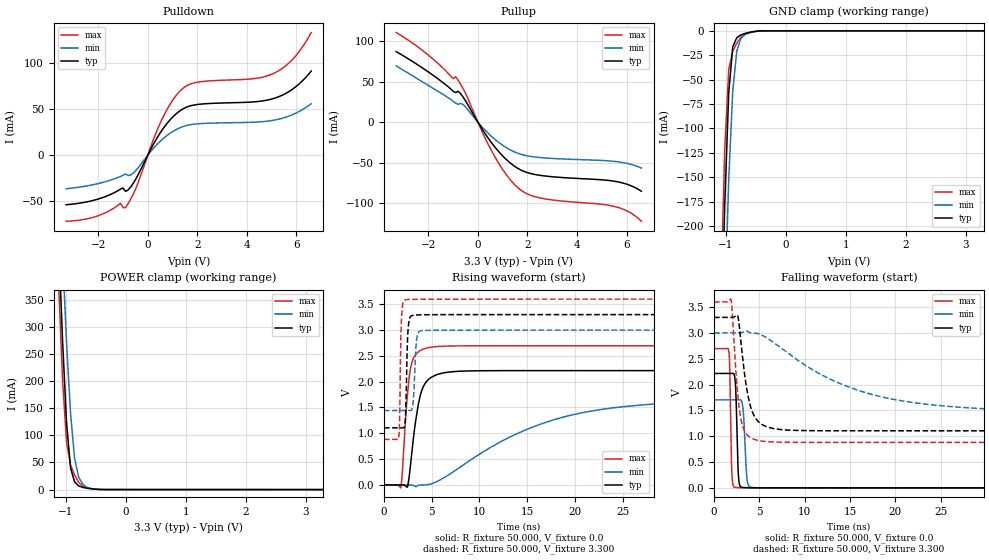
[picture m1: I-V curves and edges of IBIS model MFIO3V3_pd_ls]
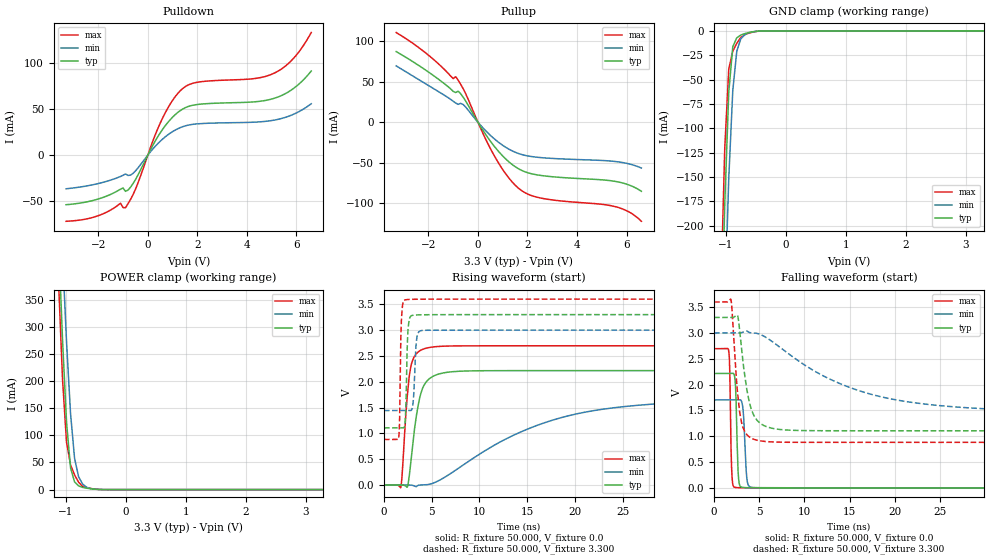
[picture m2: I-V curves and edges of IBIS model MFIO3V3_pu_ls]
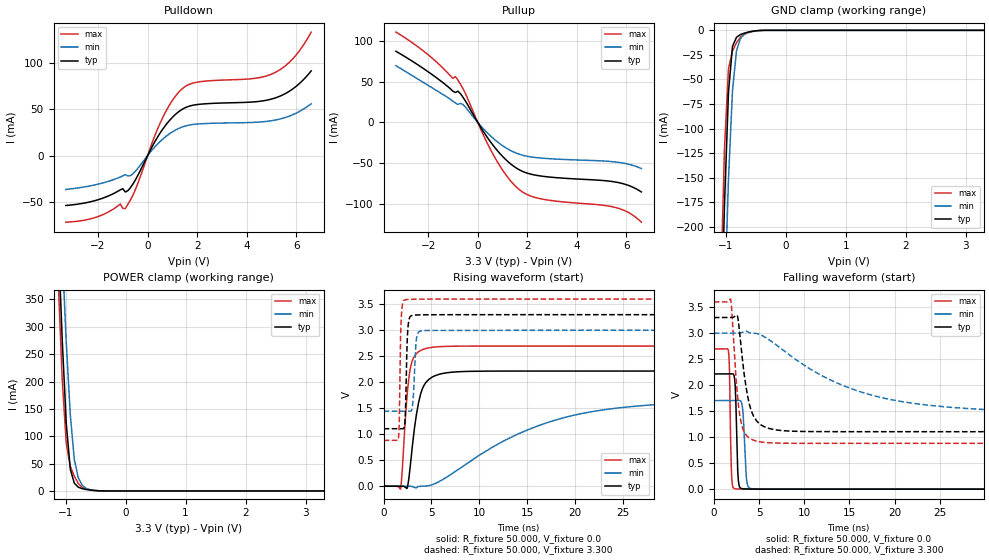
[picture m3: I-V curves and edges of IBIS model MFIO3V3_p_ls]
| IBIS file lpc55s1x_vfbga98.ibs
[IBIS Ver]   5.0
[File name]   lpc55s1x_vfbga98.ibs
[File Rev]   1.0
[Date]   June 18,2020
[Notes]   Rev History
|   1.0  initial release
[Disclaimer]   The model given below represents a 98-pin package.
[Copyright]   Copyright NXP 2020
|   Component lpc55s1x:vfbga98
[Component] lpc55s1x
[Manufacturer] NXP
[Package]
|   typ   min   max
R_pkg   0.13061   0.065508   0.30829
L_pkg   2.046e-9   9.939e-10   5.651e-9
C_pkg   3.491e-13   2.146e-13   5.779e-13
[Pin]   Signal_name   model_name   R_pin   L_pin   C_pin
N13   VBAT_DCDC   POWER   NA   NA   NA
M13   VBAT_PMU   POWER   NA   NA   NA
N8   VBUS   POWER   NA   NA   NA
A9   VDD   POWER   NA   NA   NA
A5   VDD   POWER   NA   NA   NA
M1   VDD   POWER   NA   NA   NA
A13   VDD   POWER   NA   NA   NA
G2   VDDA   POWER   NA   NA   NA
N7   USB1_3V3   POWER   NA   NA   NA
A3   USB0_3V3   POWER   NA   NA   NA
M9   VDD_PMU   POWER   NA   NA   NA
H1   VREFN   NC   NA   NA   NA
G1   VREFP   NC   NA   NA   NA
N6   USB1_DM   NC   0.11669   1.732e-9   2.843e-13
M6   USB1_DP   NC   0.11608   1.667e-9   2.908e-13
N9   FB   NC   0.1161   1.684e-9   2.591e-13
N11   LX   NC   0.065508   1.382e-9   3.314e-13
L12   P0_0   gpio3v3   0.14455   2.198e-9   3.521e-13
F5   P0_1   gpio3v3   0.090747   1.591e-9   4.4e-13
B11   P0_2   gpio3v3   0.13207   1.835e-9   3.536e-13
F8   P0_3   gpio3v3   0.10051   1.437e-9   4.428e-13
E7   P0_4   gpio3v3   0.07496   1.173e-9   3.73e-13
A7   P0_5   gpio3v3   0.14141   2.213e-9   2.521e-13
B7   P0_6   gpio3v3   0.10225   1.431e-9   2.556e-13
G5   P0_7   gpio3v3   0.14307   2.547e-9   5.485e-13
M2   P0_8   gpio3v3   0.13069   1.904e-9   2.997e-13
L13   P0_9   gpio3v3   0.16996   2.85e-9   3.914e-13
F2   P0_10   gpio3v3   0.1455   2.479e-9   3.552e-13
F1   P0_11   gpio3v3   0.12654   1.782e-9   2.328e-13
E2   P0_12   gpio3v3   0.12249   2.232e-9   2.882e-13
C12   P0_13   iicgpio3v3  0.13173   2.058e-9   2.548e-13
C13   P0_14   iicgpio3v3  0.14686   2.267e-9   2.614e-13
L2   P0_15   gpio3v3   0.11536   1.578e-9   3.074e-13
J2   P0_16   gpio3v3   0.16378   2.774e-9   3.403e-13
G3   P0_17   gpio3v3   0.076051   1.338e-9   3.659e-13
H9   P0_18   gpio3v3   0.099545   1.572e-9   4.786e-13
E6   P0_19   gpio3v3   0.10118   1.907e-9   4.333e-13
B12   P0_20   gpio3v3   0.13506   2.134e-9   3.591e-13
A12   P0_21   gpio3v3   0.14732   2.073e-9   3.225e-13
E9   P0_22   gpio3v3   0.078558   9.939e-10   3.497e-13
J1   P0_23   gpio3v3   0.13644   1.839e-9   2.161e-13
E12   P0_24   gpio3v3   0.14263   2.181e-9   2.725e-13
A11   P0_25   gpio3v3   0.14798   2.102e-9   2.79e-13
H12   P0_26   gpio3v3   0.11228   1.606e-9   2.445e-13
N2   P0_27   gpio3v3   0.16245   2.487e-9   3.312e-13
F13   P0_28   gpio3v3   0.12376   1.834e-9   2.235e-13
H8   P0_29   gpio3v3   0.13203   2.551e-9   5.469e-13
E5   P0_30   gpio3v3   0.084435   1.283e-9   4.113e-13
L1   P0_31   gpio3v3   0.14669   2.123e-9   2.715e-13
E1   P1_0   gpio3v3   0.13529   2.048e-9   2.414e-13
G11   P1_1   gpio3v3   0.074092   1.205e-9   2.789e-13
G12   P1_2   gpio3v3   0.10494   1.512e-9   2.312e-13
G13   P1_3   gpio3v3   0.12602   1.85e-9   2.146e-13
B2   P1_4   gpio3v3   0.1228   1.733e-9   2.552e-13
M5   P1_5   gpio3v3   0.13163   1.821e-9   2.471e-13
H5   P1_6   gpio3v3   0.17302   2.947e-9   5.779e-13
J5   P1_7   gpio3v3   0.13225   2.135e-9   5.089e-13
A6   P1_8   gpio3v3   0.2994   5.534e-9   4.497e-13
C1   P1_9   gpio3v3   0.15079   2.581e-9   2.461e-13
J7   P1_10   gpio3v3   0.095691   1.435e-9   3.574e-13
G6   P1_11   gpio3v3   0.12438   2.138e-9   5.286e-13
F12   P1_12   gpio3v3   0.10269   1.43e-9   2.354e-13
B3   P1_13   gpio3v3   0.096086   1.515e-9   3.876e-13
L7   P1_14   gpio3v3   0.19623   3.642e-9   4.84e-13
B6   P1_15   gpio3v3   0.17552   2.69e-9   3.435e-13
C7   P1_16   gpio3v3   0.096915   1.392e-9   2.638e-13
J9   P1_17   gpio3v3   0.092963   1.486e-9   3.448e-13
G9   P1_18   gpio3v3   0.099814   1.421e-9   3.963e-13
H13   P1_19   gpio3v3   0.13318   2.11e-9   2.391e-13
C2   P1_20   gpio3v3   0.12316   2.129e-9   3.37e-13
M7   P1_21   gpio3v3   0.11945   2.176e-9   4.385e-13
M8   P1_22   gpio3v3   0.10948   1.392e-9   2.932e-13
J8   P1_23   gpio3v3   0.075093   9.959e-10   3.672e-13
F6   P1_24   gpio3v3   0.13859   2.139e-9   5.025e-13
B8   P1_25   gpio3v3   0.21198   3.592e-9   3.673e-13
E13   P1_26   gpio3v3   0.12693   1.882e-9   2.48e-13
E8   P1_27   gpio3v3   0.097026   1.482e-9   4.012e-13
A8   P1_28   gpio3v3   0.30829   5.651e-9   4.711e-13
G8   P1_29   gpio3v3   0.1184   1.994e-9   5.418e-13
F9   P1_30   gpio3v3   0.096855   1.515e-9   4.153e-13
H6   P1_31   gpio3v3   0.15561   2.896e-9   5.731e-13
J6   RESETN   gpio3v3   0.11246   1.658e-9   3.351e-13
A1   USB0_DM   NC   0.18721   2.704e-9   3.289e-13
A2   USB0_DP   NC   0.17884   2.424e-9   3.329e-13
J12   XTAL32K_N   NC   0.11929   1.659e-9   2.629e-13
J13   XTAL32K_P   NC   0.14517   1.945e-9   2.651e-13
M3   XTAL32M_N   NC   0.13348   1.673e-9   4.297e-13
N3   XTAL32M_P   NC   0.15113   2.064e-9   4.226e-13
B13   VSS   GND   NA   NA   NA
B9   VSS   GND   NA   NA   NA
B5   VSS   GND   NA   NA   NA
N1   VSS   GND   NA   NA   NA
H2   VSSA   GND   NA   NA   NA
N5   USB1_VSS   GND   NA   NA   NA
N12   VSS_DCDC   GND   NA   NA   NA
M12   VSS_DCDC   GND   NA   NA   NA
M11   VSS_PMU   GND   NA   NA   NA
B1   USB0_VSS   GND   NA   NA   NA
|   Model Selector
[Model Selector] gpio3v3
MFIO3V3_pd_hs  EPUN=1 EPD=1 EHS=1
MFIO3V3_pd_ls  EPUN=1 EPD=1 EHS=0
MFIO3V3_pu_hs  EPUN=0 EPD=0 EHS=1
MFIO3V3_pu_ls  EPUN=0 EPD=0 EHS=0
MFIO3V3_p_hs  EPUN=1 EPD=0 EHS=1
MFIO3V3_p_ls  EPUN=1 EPD=0 EHS=0
MFIO3V3_r_hs  EPUN=0 EPD=1 EHS=1
MFIO3V3_r_ls  EPUN=0 EPD=1 EHS=0
[Model Selector] iicgpio3v3
IIC3V3_pd_hs  EGP=1 EPUN=1 EPD=1 EHS=1
IIC3V3_pd_ls  EGP=1 EPUN=1 EPD=1 EHS=0
IIC3V3_p_hs  EGP=1 EPUN=1 EPD=0 EHS=1
IIC3V3_p_ls  EGP=1 EPUN=1 EPD=0 EHS=0
IIC3V3_pu_hs  EGP=1 EPUN=0 EPD=0 EHS=1
IIC3V3_pu_ls  EGP=1 EPUN=0 EPD=0 EHS=0
IIC3V3_r_hs  EGP=1 EPUN=0 EPD=1 EHS=1
IIC3V3_r_ls  EGP=1 EPUN=0 EPD=1 EHS=0
IIC3V3_pd_iic_hs  EGP=0 ECS=0 EPUN=1 EPD=1
IIC3V3_p_iic_hs  EGP=0 ECS=0 EPUN=1 EPD=0
IIC3V3_pu_iic_hs  EGP=0 ECS=0 EPUN=0 EPD=0
IIC3V3_r_iic_hs  EGP=0 ECS=0 EPUN=0 EPD=1
IIC3V3_pd_iic_pu_hs  EGP=0 ECS=1 EPUN=1 EPD=1  SSEL=1
IIC3V3_p_iic_pu_hs  EGP=0 ECS=1 EPUN=1 EPD=0  SSEL=1
IIC3V3_pu_iic_pu_hs  EGP=0 ECS=1 EPUN=0 EPD=0  SSEL=1
IIC3V3_r_iic_pu_hs  EGP=0 ECS=1 EPUN=0 EPD=1  SSEL=1
| Models and submodels in the file (24): MFIO3V3_pd_hs (I/O), MFIO3V3_pd_ls (I/O), MFIO3V3_pu_hs (I/O), MFIO3V3_pu_ls (I/O), MFIO3V3_p_hs (I/O), MFIO3V3_p_ls (I/O), MFIO3V3_r_hs (I/O), MFIO3V3_r_ls (I/O), IIC3V3_pd_hs (I/O), IIC3V3_pd_ls (I/O), IIC3V3_p_hs (I/O), IIC3V3_p_ls (I/O), IIC3V3_pu_hs (I/O), IIC3V3_pu_ls (I/O), IIC3V3_r_hs (I/O), IIC3V3_r_ls (I/O), IIC3V3_pd_iic_hs (I/O_open_drain), IIC3V3_p_iic_hs (I/O_open_drain), IIC3V3_pu_iic_hs (I/O_open_drain), IIC3V3_r_iic_hs (I/O_open_drain), IIC3V3_pd_iic_pu_hs (I/O_open_drain), IIC3V3_p_iic_pu_hs (I/O_open_drain), IIC3V3_pu_iic_pu_hs (I/O_open_drain), IIC3V3_r_iic_pu_hs (I/O_open_drain)
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|   Model MFIO3V3_pd_ls
[Model] MFIO3V3_pd_ls
Model_type I/O
Polarity   Non-Inverting
Enable   Active-Low
Vinl =  0.990V
Vinh =  2.310V
Vmeas =  1.650V
Cref =  0.0F
Rref =  100.000
Vref =  0.0V
C_comp   1.906pF   1.877pF   1.925pF
C_comp_pullup   1.141pF   1.113pF   1.145pF
C_comp_pulldown   0.641pF   0.601pF   0.647pF
[Model Spec]
Vinh   2.310V   2.100V   2.520V
Vinl   0.990V   0.900V   1.080V
Vmeas   1.650V   1.500V   1.800V
Vref   0.0V   0.0V   0.0V
Cref   0.0F   0.0F   0.0F
Rref   100.000   100.000   100.000
[Temperature Range]   25.000   0.125k   -40.000
[Voltage Range]   3.300V   3.000V   3.600V
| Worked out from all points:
|   slope of the pulldown table from 0 to 0.495 V, typ, clamps not added: 20.7 ohm
|   slope of the pullup table from 0 to 0.495 V, typ, clamps not added: 21.4 ohm
|   GND clamp passes 1 mA (typ) near -0.56 V on its own axis
|   POWER clamp passes 1 mA (typ) near -0.53 V on its own axis
|   rising waveform, R_fixture 50.000, V_fixture 0.0: 20-80 % time 1.05ns typ, 11.9ns min, 670ps max; typ from 0 V to 2.21 V
|   rising waveform, R_fixture 50.000, V_fixture 3.300: 20-80 % time 176ps typ, 234ps min, 146ps max; typ from 1.1 V to 3.3 V
|   falling waveform, R_fixture 50.000, V_fixture 0.0: 20-80 % time 203ps typ, 279ps min, 162ps max; typ from 2.21 V to 0 V
|   falling waveform, R_fixture 50.000, V_fixture 3.300: 20-80 % time 1.13ns typ, 11.2ns min, 744ps max; typ from 3.3 V to 1.1 V
[Pulldown]
|Voltage   I(typ)   I(min)   I(max)
-3.3V     -53.7mA    -36.43mA   -71.67mA
-2.1V     -48.29mA   -31.37mA   -66.51mA
-1.1V     -36.82mA   -23.05mA   -52.1mA
-900mV    -39.2mA    -20.39mA   -56.91mA
-600mV    -30.96mA   -19.83mA   -42.97mA
600mV     28.07mA    17.5mA     40.4mA
1V        41.17mA    25.53mA    59.41mA
1.4V      49.87mA    30.79mA    72.04mA
2V        54.93mA    33.94mA    79.03mA
5V        60.84mA    37.53mA    87.68mA
5.9V      72.62mA    44.52mA    105.4mA
6.6V      91.19mA    55.78mA    132.9mA
[Pullup]
|Voltage   I(typ)   I(min)   I(max)
-3.3V     87.16mA    69.54mA    110.7mA
-2.1V     64.12mA    47.22mA    85.31mA
-1V       38.1mA     25.85mA    53.88mA
-900mV    36.64mA    23.75mA    56.16mA
-800mV    38.25mA    22.02mA    51.93mA
-600mV    31.06mA    21.93mA    41.58mA
700mV     -31.25mA   -21.55mA   -43.56mA
1.2V      -47.6mA    -32.42mA   -66.97mA
1.7V      -58.52mA   -39.3mA    -83.05mA
2.6V      -66.01mA   -43.88mA   -94.06mA
5.6V      -73.4mA    -48.74mA   -104.7mA
6.6V      -85.32mA   -56.6mA    -122.4mA
[GND_clamp]
|Voltage   I(typ)   I(min)   I(max)
-3.3V     -7.222A    -7.177A    -7.278A
-1.089V   -337.1mA   -440.8mA   -274.1mA
-1.022V   -178.2mA   -284.2mA   -121mA
-955mV    -63.05mA   -151.6mA   -39.25mA
-888mV    -16.33mA   -61.34mA   -20.9mA
-821mV    -7.066mA   -20.84mA   -12.66mA
-754mV    -4.265mA   -8.157mA   -6.693mA
-687mV    -2.794mA   -3.896mA   -3.841mA
-620mV    -1.725mA   -1.894mA   -2.339mA
-419mV    -112.4uA   -138.2uA   -135uA
3.3V      0A         0A         0A
[POWER_clamp]
|Voltage   I(typ)   I(min)   I(max)
-3.3V     8.016A     7.986A     8.074A
-1.122V   463.8mA    614.4mA    385mA
-1.055V   276.3mA    435mA      203.9mA
-988mV    124.1mA    272.4mA    87.22mA
-921mV    40.03mA    140.2mA    45.68mA
-854mV    14.24mA    57.83mA    27.12mA
-787mV    6.921mA    23.8mA     13.77mA
-720mV    4.141mA    10.27mA    6.207mA
-653mV    2.682mA    4.42mA     3.699mA
-586mV    1.616mA    1.919mA    2.191mA
-452mV    346.9uA    411.9uA    422.9uA
3.3V      0A         0A         0A
[Ramp]
| variable   typ   min   max
dV/dt_r   1.328/1.048n   1.021/11.887n   1.617/0.670n
dV/dt_f   1.317/1.132n   0.935/11.171n   1.631/0.743n
R_load = 50.000
[Rising Waveform]
R_fixture= 50.000
V_fixture= 0.0
V_fixture_min= 0.0
V_fixture_max= 0.0
|time   V(typ)   V(min)   V(max)
0s        11.38nV    124.8nV    46.5nV
1.76ns    11.77uV    -379.4nV   -52.39mV
1.89ns    124.5uV    -254.1nV   156mV
2.47ns    -34.09mV   65.71uV    1.767V
2.93ns    642.6mV    -4.824mV   2.378V
3.75ns    1.693V     -3.224mV   2.598V
4.9ns     2.078V     17.79mV    2.667V
15.38ns   2.214V     1.106V     2.695V
25.84ns   2.214V     1.529V     2.695V
100ns     2.214V     1.702V     2.695V
[Rising Waveform]
R_fixture= 50.000
V_fixture= 3.300
V_fixture_min= 3.000
V_fixture_max= 3.600
|time   V(typ)   V(min)   V(max)
0s        1.105V     1.44V      880.4mV
1.55ns    1.105V     1.44V      919.2mV
1.85ns    1.105V     1.44V      3.271V
2.2ns     1.184V     1.44V      3.582V
2.34ns    1.855V     1.44V      3.589V
2.64ns    3.192V     1.44V      3.594V
3.07ns    3.287V     1.621V     3.596V
3.43ns    3.293V     2.839V     3.597V
4.06ns    3.296V     2.992V     3.598V
100ns     3.299V     2.999V     3.599V
[Falling Waveform]
R_fixture= 50.000
V_fixture= 0.0
V_fixture_min= 0.0
V_fixture_max= 0.0
|time   V(typ)   V(min)   V(max)
0s        2.214V     1.703V     2.695V
1.63ns    2.214V     1.703V     2.64V
1.73ns    2.214V     1.703V     2.3V
1.97ns    2.214V     1.703V     263mV
2.38ns    1.941V     1.702V     7.184mV
2.7ns     199.7mV    1.703V     3.012mV
3.2ns     7.193mV    1.527V     1.541mV
3.63ns    2.938mV    178.8mV    1.008mV
4.26ns    1.462mV    6.421mV    552.8uV
100ns     15.88nV    209.7nV    49.27nV
[Falling Waveform]
R_fixture= 50.000
V_fixture= 3.300
V_fixture_min= 3.000
V_fixture_max= 3.600
|time   V(typ)   V(min)   V(max)
0s        3.299V     2.999V     3.599V
1.87ns    3.299V     2.999V     3.646V
2.6ns     3.336V     2.999V     1.836V
3.1ns     2.603V     3.009V     1.222V
3.85ns    1.693V     3.011V     992.4mV
4.41ns    1.398V     2.998V     939.4mV
5.16ns    1.242V     2.965V     908.2mV
14.39ns   1.105V     1.984V     880.4mV
25.09ns   1.105V     1.589V     880.4mV
100ns     1.105V     1.44V      880.4mV
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|   Model MFIO3V3_pu_ls
[Model] MFIO3V3_pu_ls
Model_type I/O
Polarity   Non-Inverting
Enable   Active-Low
Vinl =  0.990V
Vinh =  2.310V
Vmeas =  1.650V
Cref =  0.0F
Rref =  100.000
Vref =  0.0V
C_comp   1.906pF   1.877pF   1.925pF
C_comp_pullup   1.139pF   1.112pF   1.144pF
C_comp_pulldown   0.643pF   0.602pF   0.649pF
[Model Spec]
Vinh   2.310V   2.100V   2.520V
Vinl   0.990V   0.900V   1.080V
Vmeas   1.650V   1.500V   1.800V
Vref   0.0V   0.0V   0.0V
Cref   0.0F   0.0F   0.0F
Rref   100.000   100.000   100.000
[Temperature Range]   25.000   0.125k   -40.000
[Voltage Range]   3.300V   3.000V   3.600V
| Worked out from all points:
|   slope of the pulldown table from 0 to 0.495 V, typ, clamps not added: 20.7 ohm
|   slope of the pullup table from 0 to 0.495 V, typ, clamps not added: 21.4 ohm
|   GND clamp passes 1 mA (typ) near -0.55 V on its own axis
|   POWER clamp passes 1 mA (typ) near -0.54 V on its own axis
|   rising waveform, R_fixture 50.000, V_fixture 0.0: 20-80 % time 1.05ns typ, 11.9ns min, 674ps max; typ from 0.001 V to 2.21 V
|   rising waveform, R_fixture 50.000, V_fixture 3.300: 20-80 % time 179ps typ, 230ps min, 146ps max; typ from 1.11 V to 3.3 V
|   falling waveform, R_fixture 50.000, V_fixture 0.0: 20-80 % time 203ps typ, 278ps min, 162ps max; typ from 2.21 V to 0.001 V
|   falling waveform, R_fixture 50.000, V_fixture 3.300: 20-80 % time 1.14ns typ, 11.2ns min, 744ps max; typ from 3.3 V to 1.11 V
[Pulldown]
|Voltage   I(typ)   I(min)   I(max)
-3.3V     -53.7mA    -36.43mA   -71.67mA
-2.1V     -48.29mA   -31.37mA   -66.51mA
-1.1V     -36.82mA   -23.05mA   -52.1mA
-900mV    -39.2mA    -20.39mA   -56.91mA
-600mV    -30.96mA   -19.83mA   -42.97mA
600mV     28.07mA    17.5mA     40.4mA
1V        41.17mA    25.53mA    59.41mA
1.4V      49.87mA    30.79mA    72.04mA
2V        54.93mA    33.94mA    79.03mA
5V        60.84mA    37.53mA    87.68mA
5.9V      72.62mA    44.52mA    105.4mA
6.6V      91.19mA    55.78mA    132.9mA
[Pullup]
|Voltage   I(typ)   I(min)   I(max)
-3.3V     87.16mA    69.54mA    110.7mA
-2.1V     64.12mA    47.22mA    85.31mA
-1V       38.1mA     25.85mA    53.88mA
-900mV    36.64mA    23.75mA    56.16mA
-800mV    38.25mA    22.02mA    51.93mA
-600mV    31.06mA    21.93mA    41.58mA
700mV     -31.25mA   -21.55mA   -43.56mA
1.2V      -47.6mA    -32.42mA   -66.97mA
1.7V      -58.52mA   -39.3mA    -83.05mA
2.6V      -66.01mA   -43.88mA   -94.06mA
5.6V      -73.4mA    -48.74mA   -104.7mA
6.6V      -85.32mA   -56.6mA    -122.4mA
[GND_clamp]
|Voltage   I(typ)   I(min)   I(max)
-3.3V     -7.222A    -7.177A    -7.278A
-1.089V   -337.2mA   -440.9mA   -274.2mA
-1.022V   -178.3mA   -284.2mA   -121.1mA
-955mV    -63.12mA   -151.7mA   -39.33mA
-888mV    -16.39mA   -61.39mA   -20.98mA
-821mV    -7.132mA   -20.89mA   -12.74mA
-754mV    -4.331mA   -8.209mA   -6.777mA
-687mV    -2.86mA    -3.948mA   -3.925mA
-620mV    -1.791mA   -1.946mA   -2.423mA
-419mV    -178.1uA   -190.3uA   -219.1uA
3.3V      0A         0A         0A
[POWER_clamp]
|Voltage   I(typ)   I(min)   I(max)
-3.3V     8.016A     7.986A     8.074A
-1.122V   463.7mA    614.3mA    385mA
-1.055V   276.3mA    434.9mA    203.9mA
-988mV    124mA      272.3mA    87.13mA
-921mV    39.96mA    140.1mA    45.6mA
-854mV    14.17mA    57.77mA    27.03mA
-787mV    6.855mA    23.75mA    13.68mA
-720mV    4.075mA    10.22mA    6.123mA
-653mV    2.616mA    4.368mA    3.615mA
-586mV    1.55mA     1.867mA    2.107mA
-452mV    281.1uA    359.9uA    338.7uA
3.3V      0A         0A         0A
[Ramp]
| variable   typ   min   max
dV/dt_r   1.329/1.048n   1.022/11.881n   1.617/0.670n
dV/dt_f   1.316/1.133n   0.935/11.179n   1.631/0.744n
R_load = 50.000
[Rising Waveform]
R_fixture= 50.000
V_fixture= 0.0
V_fixture_min= 0.0
V_fixture_max= 0.0
|time   V(typ)   V(min)   V(max)
0s        869.8uV    949.2uV    842.8uV
1.76ns    883.1uV    948.8uV    -50.04mV
1.91ns    1.009mV    949.1uV    208mV
2.46ns    -36.02mV   1.012mV    1.752V
2.89ns    574.4mV    -2.122mV   2.352V
3.71ns    1.664V     -1.354mV   2.595V
4.93ns    2.083V     22.11mV    2.669V
15.41ns   2.215V     1.111V     2.696V
25.89ns   2.215V     1.532V     2.696V
100ns     2.215V     1.704V     2.696V
[Rising Waveform]
R_fixture= 50.000
V_fixture= 3.300
V_fixture_min= 3.000
V_fixture_max= 3.600
|time   V(typ)   V(min)   V(max)
0s        1.106V     1.442V     881.7mV
1.55ns    1.106V     1.442V     920.7mV
1.83ns    1.106V     1.442V     3.201V
2.2ns     1.19V      1.442V     3.584V
2.36ns    2.014V     1.442V     3.591V
2.67ns    3.219V     1.441V     3.595V
3.05ns    3.288V     1.591V     3.597V
3.47ns    3.295V     2.885V     3.598V
4.05ns    3.297V     2.994V     3.599V
100ns     3.3V       3V         3.6V
[Falling Waveform]
R_fixture= 50.000
V_fixture= 0.0
V_fixture_min= 0.0
V_fixture_max= 0.0
|time   V(typ)   V(min)   V(max)
0s        2.215V     1.704V     2.696V
1.63ns    2.215V     1.704V     2.641V
1.73ns    2.215V     1.704V     2.3V
1.97ns    2.216V     1.704V     265.9mV
2.37ns    1.988V     1.704V     8.752mV
2.68ns    252.6mV    1.704V     4.211mV
3.22ns    8.138mV    1.493V     2.448mV
3.64ns    3.966mV    165.1mV    1.883mV
4.28ns    2.4mV      8.68mV     1.408mV
100ns     869.8uV    949.4uV    842.8uV
[Falling Waveform]
R_fixture= 50.000
V_fixture= 3.300
V_fixture_min= 3.000
V_fixture_max= 3.600
|time   V(typ)   V(min)   V(max)
0s        3.3V       3V         3.6V
1.88ns    3.3V       3V         3.639V
2.61ns    3.334V     3V         1.817V
3.06ns    2.664V     3.008V     1.251V
3.83ns    1.711V     3.015V     996.5mV
4.37ns    1.414V     3.001V     943.5mV
5.06ns    1.258V     2.975V     912.3mV
14.38ns   1.106V     1.987V     881.7mV
25.08ns   1.106V     1.591V     881.7mV
100ns     1.106V     1.442V     881.7mV
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|   Model MFIO3V3_p_ls
[Model] MFIO3V3_p_ls
Model_type I/O
Polarity   Non-Inverting
Enable   Active-Low
Vinl =  0.990V
Vinh =  2.310V
Vmeas =  1.650V
Cref =  0.0F
Rref =  100.000
Vref =  0.0V
C_comp   1.906pF   1.877pF   1.925pF
C_comp_pullup   1.140pF   1.112pF   1.144pF
C_comp_pulldown   0.642pF   0.602pF   0.649pF
[Model Spec]
Vinh   2.310V   2.100V   2.520V
Vinl   0.990V   0.900V   1.080V
Vmeas   1.650V   1.500V   1.800V
Vref   0.0V   0.0V   0.0V
Cref   0.0F   0.0F   0.0F
Rref   100.000   100.000   100.000
[Temperature Range]   25.000   0.125k   -40.000
[Voltage Range]   3.300V   3.000V   3.600V
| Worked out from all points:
|   slope of the pulldown table from 0 to 0.495 V, typ, clamps not added: 20.7 ohm
|   slope of the pullup table from 0 to 0.495 V, typ, clamps not added: 21.4 ohm
|   GND clamp passes 1 mA (typ) near -0.56 V on its own axis
|   POWER clamp passes 1 mA (typ) near -0.54 V on its own axis
|   rising waveform, R_fixture 50.000, V_fixture 0.0: 20-80 % time 1.05ns typ, 11.9ns min, 670ps max; typ from 0 V to 2.21 V
|   rising waveform, R_fixture 50.000, V_fixture 3.300: 20-80 % time 177ps typ, 237ps min, 147ps max; typ from 1.1 V to 3.3 V
|   falling waveform, R_fixture 50.000, V_fixture 0.0: 20-80 % time 203ps typ, 282ps min, 162ps max; typ from 2.21 V to 0 V
|   falling waveform, R_fixture 50.000, V_fixture 3.300: 20-80 % time 1.14ns typ, 11.2ns min, 740ps max; typ from 3.3 V to 1.1 V
[Pulldown]
|Voltage   I(typ)   I(min)   I(max)
-3.3V     -53.7mA    -36.43mA   -71.67mA
-2.1V     -48.29mA   -31.37mA   -66.51mA
-1.1V     -36.82mA   -23.05mA   -52.1mA
-900mV    -39.2mA    -20.39mA   -56.91mA
-600mV    -30.96mA   -19.83mA   -42.97mA
600mV     28.07mA    17.5mA     40.4mA
1V        41.17mA    25.53mA    59.41mA
1.4V      49.87mA    30.79mA    72.04mA
2V        54.93mA    33.94mA    79.03mA
5V        60.84mA    37.53mA    87.68mA
5.9V      72.62mA    44.52mA    105.4mA
6.6V      91.19mA    55.78mA    132.9mA
[Pullup]
|Voltage   I(typ)   I(min)   I(max)
-3.3V     87.16mA    69.54mA    110.7mA
-2.1V     64.12mA    47.22mA    85.31mA
-1V       38.1mA     25.85mA    53.88mA
-900mV    36.64mA    23.75mA    56.16mA
-800mV    38.25mA    22.02mA    51.93mA
-600mV    31.06mA    21.93mA    41.58mA
700mV     -31.25mA   -21.55mA   -43.56mA
1.2V      -47.6mA    -32.42mA   -66.97mA
1.7V      -58.52mA   -39.3mA    -83.05mA
2.6V      -66.01mA   -43.88mA   -94.06mA
5.6V      -73.4mA    -48.74mA   -104.7mA
6.6V      -85.32mA   -56.6mA    -122.4mA
[GND_clamp]
|Voltage   I(typ)   I(min)   I(max)
-3.3V     -7.222A    -7.177A    -7.278A
-1.089V   -337.1mA   -440.8mA   -274.1mA
-1.022V   -178.2mA   -284.2mA   -121mA
-955mV    -63.04mA   -151.6mA   -39.24mA
-888mV    -16.32mA   -61.33mA   -20.89mA
-821mV    -7.057mA   -20.83mA   -12.64mA
-754mV    -4.256mA   -8.15mA    -6.682mA
-687mV    -2.785mA   -3.888mA   -3.83mA
-620mV    -1.717mA   -1.887mA   -2.329mA
-419mV    -104.8uA   -131.8uA   -126uA
3.3V      0A         0A         0A
[POWER_clamp]
|Voltage   I(typ)   I(min)   I(max)
-3.3V     8.016A     7.986A     8.074A
-1.122V   463.7mA    614.3mA    384.9mA
-1.055V   276.2mA    434.9mA    203.8mA
-988mV    124mA      272.3mA    87.12mA
-921mV    39.95mA    140.1mA    45.59mA
-854mV    14.16mA    57.77mA    27.02mA
-787mV    6.846mA    23.74mA    13.67mA
-720mV    4.066mA    10.21mA    6.113mA
-653mV    2.607mA    4.361mA    3.605mA
-586mV    1.542mA    1.86mA     2.097mA
-452mV    273.4uA    353.7uA    329.6uA
3.3V      0A         0A         0A
[Ramp]
| variable   typ   min   max
dV/dt_r   1.329/1.049n   1.022/11.884n   1.618/0.670n
dV/dt_f   1.317/1.134n   0.935/11.178n   1.632/0.744n
R_load = 50.000
[Rising Waveform]
R_fixture= 50.000
V_fixture= 0.0
V_fixture_min= 0.0
V_fixture_max= 0.0
|time   V(typ)   V(min)   V(max)
0s        11.91nV    127.2nV    48.18nV
1.76ns    14.07uV    -353.2nV   -52.48mV
1.9ns     130.3uV    -106.1nV   185.6mV
2.46ns    -38.99mV   62.57uV    1.761V
2.93ns    644.9mV    -4.797mV   2.378V
3.65ns    1.606V     -5.408mV   2.586V
4.94ns    2.084V     20.24mV    2.669V
15.63ns   2.215V     1.125V     2.696V
25.83ns   2.215V     1.53V      2.696V
100ns     2.215V     1.703V     2.696V
[Rising Waveform]
R_fixture= 50.000
V_fixture= 3.300
V_fixture_min= 3.000
V_fixture_max= 3.600
|time   V(typ)   V(min)   V(max)
0s        1.105V     1.441V     880.7mV
1.55ns    1.105V     1.441V     919.6mV
1.84ns    1.105V     1.441V     3.233V
2.22ns    1.224V     1.441V     3.584V
2.37ns    2.139V     1.441V     3.59V
2.68ns    3.224V     1.44V      3.594V
3.06ns    3.287V     1.603V     3.596V
3.45ns    3.294V     2.861V     3.598V
4.07ns    3.297V     2.993V     3.599V
100ns     3.3V       3V         3.6V
[Falling Waveform]
R_fixture= 50.000
V_fixture= 0.0
V_fixture_min= 0.0
V_fixture_max= 0.0
|time   V(typ)   V(min)   V(max)
0s        2.215V     1.703V     2.696V
1.62ns    2.215V     1.703V     2.651V
1.73ns    2.215V     1.703V     2.303V
1.97ns    2.215V     1.703V     265.7mV
2.37ns    1.981V     1.703V     8.251mV
2.69ns    225.2mV    1.704V     3.621mV
3.22ns    7.595mV    1.492V     1.863mV
3.64ns    3.369mV    166.1mV    1.261mV
4.27ns    1.779mV    7.484mV    732uV
100ns     16.41nV    212.2nV    50.94nV
[Falling Waveform]
R_fixture= 50.000
V_fixture= 3.300
V_fixture_min= 3.000
V_fixture_max= 3.600
|time   V(typ)   V(min)   V(max)
0s        3.3V       3V         3.6V
1.88ns    3.3V       3V         3.641V
2.61ns    3.334V     3V         1.821V
3.08ns    2.642V     3.009V     1.24V
3.83ns    1.711V     3.015V     995.8mV
4.38ns    1.41V      3.001V     942.3mV
5.17ns    1.242V     2.968V     908.5mV
14.42ns   1.105V     1.984V     880.8mV
25.12ns   1.105V     1.59V      880.7mV
100ns     1.105V     1.441V     880.7mV
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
